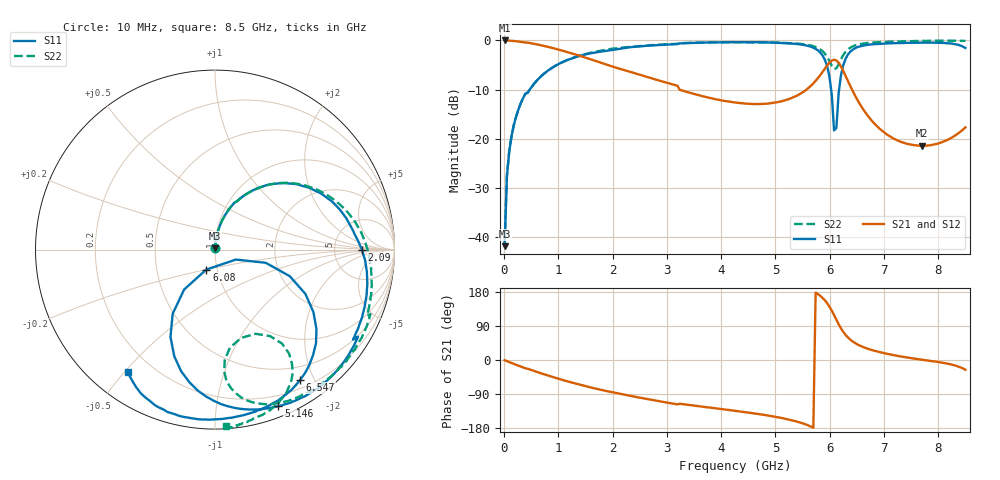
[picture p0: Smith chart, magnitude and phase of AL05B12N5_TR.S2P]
!AVX Corporation
!PN: AL05B12N5*TR
!Description: Air Core Inductor, 12.5nH, 10 Turns
!Agilent Technologies,E5071C,MY46102230,A.09.54
!Date: Mon Sep 03 16:24:13 2012
!Data & Calibration Information:
!Freq	S11:SOLT2(ON)	S21:SOLT2(ON)	S12:SOLT2(ON)	S22:SOLT2(ON)
# Hz S dB R 50
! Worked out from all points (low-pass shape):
!   201 points, 10 MHz to 8.5 GHz, reference 50 ohm
!   highest |S21| = -0.01 dB at 10 MHz (marker M1); lowest = -21.4 dB at 7.693 GHz (marker M2)
!   |S21| within 3 dB of the highest: start of sweep to 1.357 GHz
!   lowest |S11| = -41.9 dB at 10 MHz (marker M3), VSWR 1.02, Z = 50.1 + j0.803 ohm
!   |S11| at or under -10 dB: start of sweep to 473.1 MHz; 6.026 GHz to 6.173 GHz (147.4 MHz wide, 2.42 % of centre)
!   |S22| runs from -41.4 to 0.0 dB; largest |S21 - S12| = 0.009
!   S11 on the Smith chart (normalised r, x): 10 MHz: 1.00, +0.02; 2.09 GHz: 10, +0; 5.146 GHz: 0.10, -1.48; 6.08 GHz: 0.89, -0.20; 6.547 GHz: 0.31, -1.81; 8.5 GHz: 0.11, -0.51
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1e7  -41.88 85.2  -0.01 -0.6  -0.08 -0.6  -41.40 83.8
5.245e7  -27.66 85.4  -0.02 -3.0  0.01 -3.2  -27.56 85.0
9.49e7  -22.65 83.0  -0.04 -5.5  -0.03 -5.4  -22.61 82.7
3.0715e8  -12.82 71.4  -0.28 -17.2  -0.26 -17.3  -12.78 71.7
8.59e8  -5.76 45.8  -1.45 -43.2  -1.44 -43.2  -5.76 46.0
1.4533e9  -2.97 21.3  -3.34 -67.3  -3.33 -67.3  -2.91 23.2
2.09005e9  -1.74 0.0  -5.63 -87.7  -5.63 -87.8  -1.56 3.3
2.85415e9  -0.92 -23.8  -8.16 -108.8  -8.15 -108.8  -0.86 -15.9
4.255e9  -0.35 -49.7  -12.64 -134.0  -12.65 -134.0  -0.38 -41.1
5.14645e9  -0.53 -68.0  -12.29 -154.0  -12.30 -154.0  -0.50 -59.9
5.6983e9  -1.48 -90.3  -8.74 -178.8  -8.74 -178.9  -1.17 -76.4
5.953e9  -5.25 -117.0  -5.11 149.9  -5.11 149.9  -3.37 -85.7
6.0379e9  -11.02 -127.7  -4.09 130.3  -4.10 130.2  -5.15 -81.3
6.08035e9  -18.32 -113.5  -3.93 118.6  -3.93 118.6  -5.80 -73.6
6.1228e9  -17.81 -25.6  -4.07 106.2  -4.07 106.2  -5.67 -64.2
6.16525e9  -10.69 -14.6  -4.55 94.3  -4.55 94.3  -4.86 -57.5
6.25015e9  -5.02 -26.1  -6.23 74.1  -6.23 74.1  -2.96 -54.5
6.5473e9  -1.24 -56.8  -12.81 38.4  -12.80 38.4  -0.79 -66.4
7.09915e9  -0.59 -78.7  -19.46 15.2  -19.47 15.1  -0.25 -77.9
7.69345e9  -0.45 -94.1  -21.45 0.9  -21.45 0.8  -0.10 -83.1
8.2453e9  -0.63 -111.0  -19.82 -11.9  -19.82 -11.8  -0.06 -85.5
8.5e9  -1.53 -125.5  -17.70 -25.8  -17.69 -25.7  -0.11 -86.5
